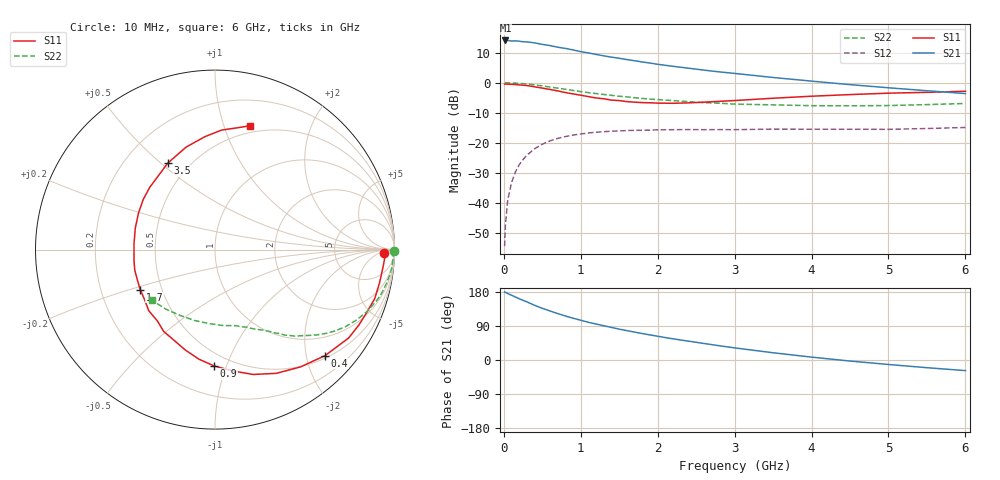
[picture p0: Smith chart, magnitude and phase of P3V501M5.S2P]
! SIEMENS Small Signal Semiconductors
! BFP181
! Si NPN RF Bipolar Junction Transistor in SOT143
! VCE = 0.5 V  IC = 1.5 mA
! Common Emitter S-Parameters:  March  1996
# GHz  S  MA  R  50
!  f  S11  S21  S12  S22
! GHz  MAG  ANG  MAG  ANG  MAG  ANG  MAG  ANG
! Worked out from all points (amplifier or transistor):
!   36 points, 10 MHz to 6 GHz, reference 50 ohm
!   highest |S21| = 14.0 dB at 20 MHz (marker M1)
!   |S21| within 3 dB of that: start of sweep to 870.1 MHz
!   unconditionally stable (mu >= 1): 2.306 GHz to end of sweep
!   at 250 MHz: K = 0.13, MSG = 19.6 dB, |S12| = -25.6 dB
!   at 1.4 GHz: K = 0.66, MSG = 12.3 dB, |S12| = -16.2 dB
!   at 6 GHz: K = 1.43, MAG = 1.7 dB, |S12| = -14.9 dB
!   S11 on the Smith chart (normalised r, x): 10 MHz: 29, -11; 400 MHz: 0.55, -2.37; 900 MHz: 0.41, -0.91; 1.7 GHz: 0.38, -0.22; 3.5 GHz: 0.38, +0.53; 6 GHz: 0.43, +1.23
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0.01  0.9424 -1.3  4.963 179.4  0.0019 86.9  0.9946 -0.5
0.02  0.9478 -2.3  5.023 178.8  0.0042 85.1  0.9932 -1.1
0.05  0.9422 -5.4  5.02 175.5  0.011 86.6  0.9925 -3.0
0.1  0.9355 -11.4  4.914 170.9  0.0217 82.7  0.9904 -5.9
0.15  0.9308 -17.1  4.942 166.3  0.0325 79.3  0.9817 -8.7
0.2  0.9147 -22.7  4.882 161.6  0.0431 75.7  0.9727 -11.5
0.3  0.8926 -33.5  4.754 153.4  0.062 68.9  0.9486 -16.9
0.4  0.8516 -43.9  4.584 144.3  0.0794 62.5  0.9158 -22.0
0.5  0.8088 -53.9  4.317 136.4  0.0944 56.5  0.8804 -26.5
0.6  0.7696 -63.6  4.127 129.4  0.1073 51.2  0.8441 -30.6
0.8  0.6827 -81.8  3.706 116.1  0.1264 42.2  0.7741 -37.1
0.9  0.6483 -90.4  3.494 110.2  0.1342 38.2  0.74 -40.0
1.1  0.5837 -106.4  3.116 99.4  0.145 31.5  0.6808 -44.8
1.3  0.5382 -122.1  2.785 90.3  0.1525 25.7  0.634 -49.0
1.5  0.5023 -137.3  2.537 81.4  0.1569 21.5  0.5927 -52.2
1.7  0.4724 -151.9  2.311 73.6  0.1604 17.8  0.5605 -55.3
2.2  0.4525 175.8  1.865 55.8  0.1646 10.9  0.5008 -62.5
2.8  0.4876 145.1  1.508 37.6  0.1653 5.5  0.4535 -71.5
3.5  0.5493 118.6  1.216 19.1  0.1682 1.2  0.4258 -83.8
4.5  0.6316 95.1  0.925 -2.8  0.1674 -3.8  0.4112 -106.4
5.5  0.6884 80.0  0.732 -20.3  0.1723 -4.5  0.4302 -129.5
6  0.7177 74.1  0.657 -28.0  0.1791 -5.6  0.4496 -141.0
